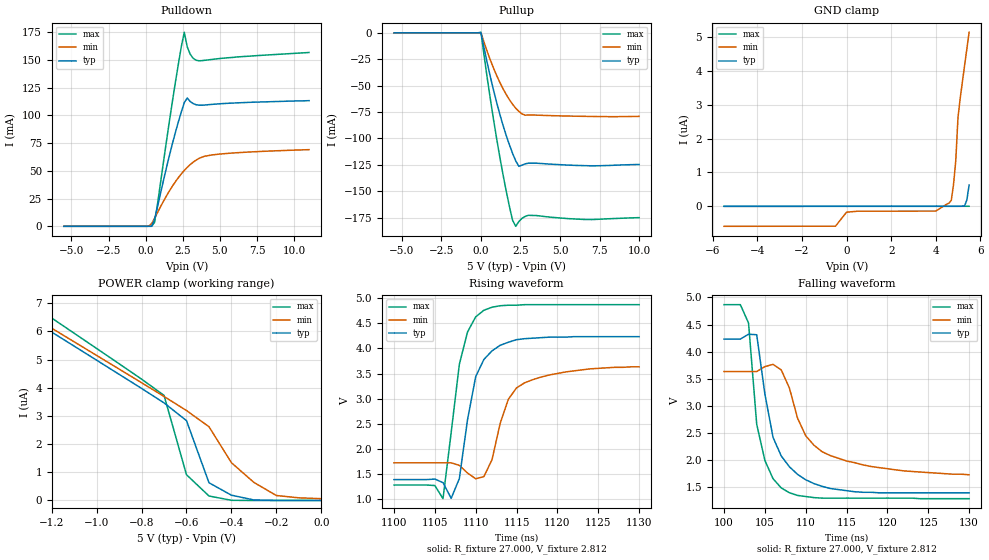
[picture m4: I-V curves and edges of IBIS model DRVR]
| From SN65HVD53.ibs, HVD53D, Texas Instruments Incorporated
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|   Driver Output / Receiver Input Model
[Model]   DRVR
Model_type   I/O
| Signals   Y,Z
Vinl = 0.9V
Vinh = 2.8V
Vmeas = 1.7V   |Reference voltage for timing measurements
Cref = 50pF   |Timing specification test load capacitance value
Rref = 54   |Note: 54 Ohm load; single-ended configuration
|   Timing specification test load voltage
| variable   typ   min   max
C_comp   28pF   24pF   32pF
|   typ   min   max
[Temperature Range]   25.0   -40   85
[Voltage range]   5.0V   4.5V   5.5V
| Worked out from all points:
|   slope of the pulldown table from 0 to 0.75 V, typ, clamps not added: 50.7 ohm
|   slope of the pullup table from 0 to 0.75 V, typ, clamps not added: 14.5 ohm
|   rising waveform, R_fixture 27.000, V_fixture 2.812: 20-80 % time 2.2ns typ, 2.92ns min, 1.98ns max; typ from 1.4 V to 4.23 V
|   falling waveform, R_fixture 27.000, V_fixture 2.812: 20-80 % time 2.98ns typ, 4.49ns min, 1.78ns max; typ from 4.23 V to 1.4 V
[Pulldown]
|   Voltage   I(typ)   I(min)   I(max)
-5.5V     -10.66pA   -1.61nA    -2.66pA
200mV     102.2nA    81.88uA    446.1pA
400mV     121.7uA    2.397mA    2.576uA
600mV     6.248mA    7.209mA    3.471mA
1.8V      74.35mA    36.14mA    112.4mA
2.4V      103mA      47.21mA    161.8mA
2.6V      111.4mA    50.31mA    174.8mA
2.8V      115.6mA    53.11mA    161.7mA
3V        112.4mA    55.6mA     155mA
3.6V      109.1mA    61.2mA     149.1mA
5.5V      110.8mA    65.68mA    151.8mA
11V       113.2mA    69.05mA    156.6mA
[Pullup]
|   Voltage   I(typ)   I(min)   I(max)
| Note that the[Pullup]voltage table is referenced to Vcc
| and is calculated using Vtable=Vcc - Vmeasured.
-5.5V     2.4uA      2.144uA    2.981uA
0V        269.5uA    177uA      535.4uA
600mV     -42.03mA   -26mA      -63.31mA
1.2V      -77.48mA   -47.12mA   -118.3mA
1.6V      -97.35mA   -58.48mA   -150.1mA
2V        -114.2mA   -67.65mA   -177.6mA
2.2V      -121.3mA   -71.41mA   -183.3mA
2.4V      -126.5mA   -74.49mA   -178.7mA
2.8V      -124.1mA   -78.04mA   -173.9mA
3V        -123.5mA   -77.81mA   -172.9mA
6.5V      -125.8mA   -79.1mA    -176.8mA
10V       -124.7mA   -79.14mA   -175.1mA
[GND_clamp]
|   Voltage  I(typ)   I(min)   I(max)
| Outputs in High Impedance (off)
-5.5V     -1.17nA    -592nA     -1.094nA
-500mV    -651.3pA   -589.2nA   -574.5pA
0V        -526.7pA   -174.9nA   -522.6pA
4V        256.2pA    -142.8nA   173.6pA
4.6V      361.5pA    94.35nA    277.1pA
4.7V      380.1pA    176.4nA    294pA
4.8V      394.4pA    641.3nA    311.8pA
4.9V      418.3pA    1.34uA     326.9pA
5V        446.8pA    2.618uA    343.7pA
5.3V      18.21nA    4.177uA    389pA
5.4V      188.2nA    4.662uA    400.6pA
5.5V      629.7nA    5.145uA    417.4pA
[POWER_clamp]
|   Voltage  I(typ)   I(min)   I(max)
| Note that the [POWER_clamp] voltage table is referenced to Vcc
| and is calculated using Vtable = Vcc - Vmeasured.
| Outputs in Tri-state.
-5.5V     27.39uA    26.86uA    29.68uA
-1.5V     7.468uA    7.559uA    8.092uA
-1.4V     6.97uA     7.077uA    7.552uA
-1.3V     6.472uA    6.594uA    7.012uA
-800mV    3.975uA    4.177uA    4.305uA
-700mV    3.462uA    3.69uA     3.728uA
-600mV    2.832uA    3.19uA     913.7nA
-500mV    629.7nA    2.618uA    159.9nA
-400mV    188.2nA    1.34uA     5.888nA
-300mV    18.21nA    641.3nA    839.3pA
-200mV    1.35nA     176.4nA    418.3pA
0V        446.8pA    64.16nA    417.4pA
[Ramp]
|   typ   min   max
dV/dt_r   1.69V/2.2ns   1.12V/2.9ns   2.14V/2.0ns
dV/dt_f   1.70V/4.2ns   1.13V/4.7ns   2.16V/2.2ns
R_load = 27ohm | Note: The measurement is on a single-ended configuration
|   with 54ohm line-to-line.
[Rising Waveform]
R_fixture = 27.000
V_fixture = 2.812
V_fixture_min = 2.663
V_fixture_max = 3.070
C_fixture = 0.000
L_fixture = 0.000
|  time   V(typ)   V(min)   V(max)
1.1us     1.395V     1.728V     1.287V
1.105us   1.405V     1.728V     1.277V
1.106us   1.335V     1.728V     1.016V
1.107us   1.023V     1.728V     2.33V
1.108us   1.415V     1.677V     3.683V
1.11us    3.438V     1.412V     4.625V
1.111us   3.779V     1.453V     4.756V
1.114us   4.121V     2.991V     4.856V
1.115us   4.172V     3.215V     4.856V
1.13us    4.232V     3.633V     4.867V
[Falling Waveform]
R_fixture = 27.000
V_fixture = 2.812
V_fixture_min = 2.663
V_fixture_max = 3.070
C_fixture = 0.000
L_fixture = 0.000
|  time   V(typ)   V(min)   V(max)
100ns     4.232V     3.633V     4.867V
102ns     4.232V     3.633V     4.867V
103ns     4.322V     3.633V     4.528V
104ns     4.312V     3.633V     2.659V
105ns     3.22V      3.724V     1.993V
106ns     2.418V     3.765V     1.655V
107ns     2.076V     3.664V     1.486V
110ns     1.636V     2.448V     1.327V
112ns     1.515V     2.154V     1.297V
130ns     1.395V     1.728V     1.287V
